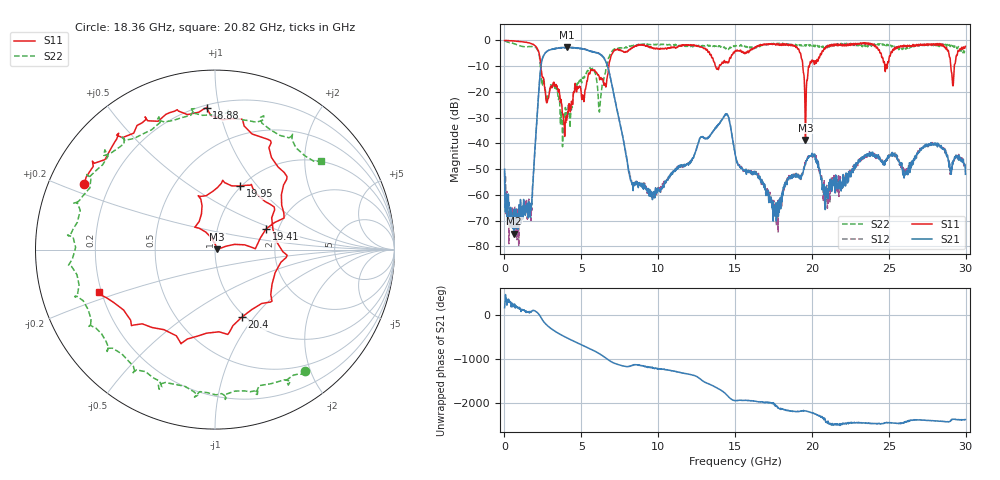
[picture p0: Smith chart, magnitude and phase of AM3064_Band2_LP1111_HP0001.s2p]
# Hz S DB R 50.0
!freq dBS11 angS11 dBS21 angS21 dBS12 angS12 dBS22 angS22
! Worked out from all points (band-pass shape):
!   1600 points, 10 MHz to 29.98 GHz, reference 50 ohm
!   highest |S21| = -2.66 dB at 4.059 GHz (marker M1); lowest = -75.1 dB at 628.5 MHz (marker M2)
!   |S21| within 3 dB of the highest: 2.569 GHz to 6.268 GHz (3.699 GHz wide, 83.7 % of centre)
!   lowest |S11| = -38.7 dB at 19.58 GHz (marker M3), VSWR 1.02, Z = 51.2 + j0.268 ohm
!   |S11| at or under -10 dB: 2.37 GHz to 6.785 GHz (4.414 GHz wide, 96.4 % of centre); 13.72 GHz to 13.98 GHz (257.9 MHz wide, 1.86 % of centre); 19.41 GHz to 19.83 GHz (426.5 MHz wide, 2.17 % of centre)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
!   |S22| runs from -41.3 to -0.1 dB; largest |S21 - S12| = 0.024
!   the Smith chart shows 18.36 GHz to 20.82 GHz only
!   S11 on the Smith chart (normalised r, x): 18.36 GHz: 0.11, +0.23; 18.88 GHz: 0.22, +0.92; 19.41 GHz: 1.73, +0.44; 19.95 GHz: 0.99, +0.82; 20.4 GHz: 0.96, -0.87; 20.82 GHz: 0.19, -0.17
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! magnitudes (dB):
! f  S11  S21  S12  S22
! 10 MHz  0.0  -50.0  -50.9  -0.1
! 628.5 MHz  -0.2  -75.1  -72.6  -1.3
! 1.697 GHz  -1.2  -63.4  -68.5  -2.4
! 2.522 GHz  -14.4  -6.2  -6.2  -14.9
! 4.059 GHz  -29.9  -2.7  -2.7  -29.8
! 5.015 GHz  -22.0  -3.2  -3.2  -16.4
! 6.627 GHz  -17.1  -8.7  -8.7  -10.2
! 8.295 GHz  -2.9  -56.0  -55.4  -2.1
! 10 GHz  -3.3  -57.4  -57.1  -1.6
! 14.39 GHz  -8.6  -28.9  -28.7  -3.3
! 15 GHz  -4.2  -44.4  -44.4  -2.1
! 17.59 GHz  -1.3  -68.3  -65.4  -1.2
! 18.36 GHz  -1.8  -55.5  -55.5  -1.5
! 18.88 GHz  -2.0  -52.7  -52.0  -2.1
! 19.41 GHz  -10.2  -51.5  -51.1  -1.7
! 19.58 GHz  -38.7  -48.2  -48.1  -2.0
! 19.95 GHz  -8.4  -44.9  -44.5  -2.1
! 19.99 GHz  -7.8  -45.0  -44.7  -1.6
! 20.4 GHz  -7.8  -47.5  -47.0  -2.5
! 20.82 GHz  -3.2  -59.2  -61.8  -2.3
! 25 GHz  -7.9  -45.6  -44.6  -1.7
! 29.98 GHz  -2.3  -52.0  -49.3  -4.3
